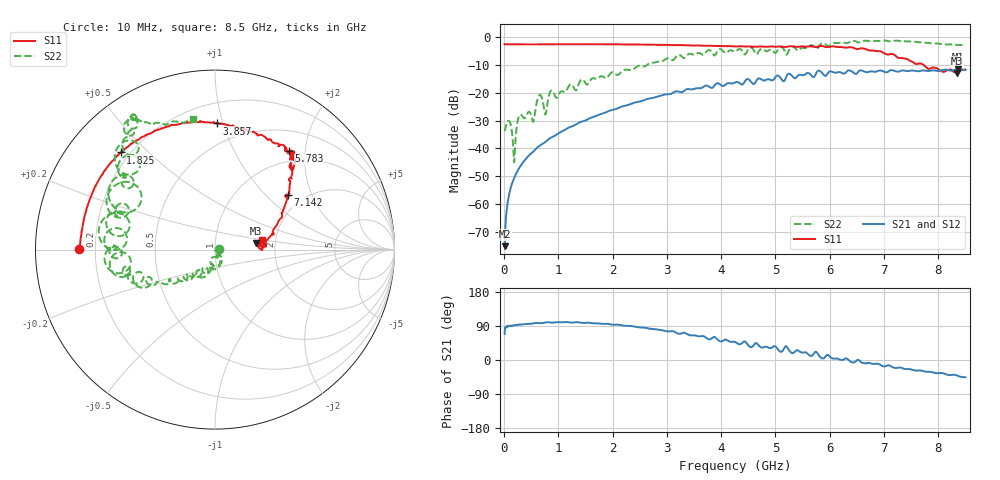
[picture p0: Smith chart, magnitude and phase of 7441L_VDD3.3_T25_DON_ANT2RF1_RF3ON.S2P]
!Agilent Technologies,E5071C,MY46417908,A.11.23
!Date: Mon May 03 19:54:17 2021
!Data & Calibration Information:
!Freq	S11:SOLT2(ON)	S21:SOLT2(ON)	S12:SOLT2(ON)	S22:SOLT2(ON)
!PortZ  Port1:50+j0  Port2:50+j0
!Above PortZ is port z conversion or system Z0 setting when saving the data.
!When reading, reference impedance value at option line is always used.
# Hz S dB R 50
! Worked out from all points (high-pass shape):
!   1601 points, 10 MHz to 8.5 GHz, reference 50 ohm
!   highest |S21| = -11.37 dB at 8.367 GHz (marker M1); lowest = -75.2 dB at 10 MHz (marker M2)
!   |S21| within 3 dB of the highest: 5.196 GHz to 5.33 GHz (134.3 MHz wide, 2.55 % of centre); 5.387 GHz to end of sweep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
!   lowest |S11| = -12.8 dB at 8.346 GHz (marker M3), VSWR 1.59, Z = 79 + j5.84 ohm
!   |S11| at or under -10 dB: 7.737 GHz to end of sweep
!   |S22| runs from -45.0 to -1.1 dB; largest |S21 - S12| = 0.0076
!   S11 on the Smith chart (normalised r, x): 10 MHz: 0.14, +0.00; 1.825 GHz: 0.16, +0.41; 3.857 GHz: 0.34, +0.95; 5.783 GHz: 0.82, +1.69; 7.142 GHz: 1.66, +1.36; 8.5 GHz: 1.69, +0.18
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1e7  -2.43 179.6  -75.24 68.8  -75.68 79.8  -33.81 2.6
9.49e7  -2.48 177.2  -56.44 89.8  -56.42 90.2  -30.12 -42.6
1.851062e8  -2.50 174.6  -50.70 92.0  -50.73 90.9  -45.01 -42.3
3.124562e8  -2.52 171.0  -46.06 93.7  -46.05 93.6  -27.82 -54.7
5.300125e8  -2.50 165.1  -41.26 96.1  -41.26 96.1  -30.24 -77.0
6.520562e8  -2.49 161.9  -39.06 97.5  -39.06 97.4  -20.75 -81.0
7.634875e8  -2.48 158.9  -37.64 99.0  -37.65 99.1  -27.80 -88.7
8.643062e8  -2.47 156.3  -36.12 98.9  -36.11 98.9  -19.21 -89.4
9.757375e8  -2.45 153.4  -34.93 99.8  -34.94 99.9  -21.71 -101.3
1.426769e9  -2.43 143.2  -30.34 98.0  -30.34 98.0  -15.13 -118.3
1.824738e9  -2.45 134.1  -27.39 95.3  -27.38 95.4  -14.13 -135.2
2.843538e9  -2.66 112.2  -21.22 79.8  -21.24 80.0  -8.70 -150.5
3.857031e9  -3.06 89.2  -17.81 60.5  -17.83 60.1  -6.22 -176.7
4.255e9  -3.23 78.1  -16.21 47.7  -16.20 47.2  -5.16 179.3
5.671769e9  -3.25 51.9  -13.86 11.2  -13.83 10.6  -2.79 135.0
5.7832e9  -3.28 53.2  -12.01 15.6  -11.99 15.2  -3.68 140.0
6.451788e9  -3.86 46.6  -12.89 -6.4  -12.93 -7.2  -1.25 123.5
7.088538e9  -6.13 37.3  -12.13 -13.9  -12.14 -14.3  -1.37 121.3
7.1416e9  -5.91 37.1  -11.77 -17.8  -11.73 -18.2  -1.28 122.6
8.346119e9  -12.79 8.8  -11.39 -40.8  -11.43 -40.9  -2.72 104.5
8.367344e9  -12.68 6.5  -11.37 -42.1  -11.41 -42.1  -2.75 104.0
8.5e9  -11.53 11.0  -11.66 -45.5  -11.68 -45.4  -2.62 99.7
